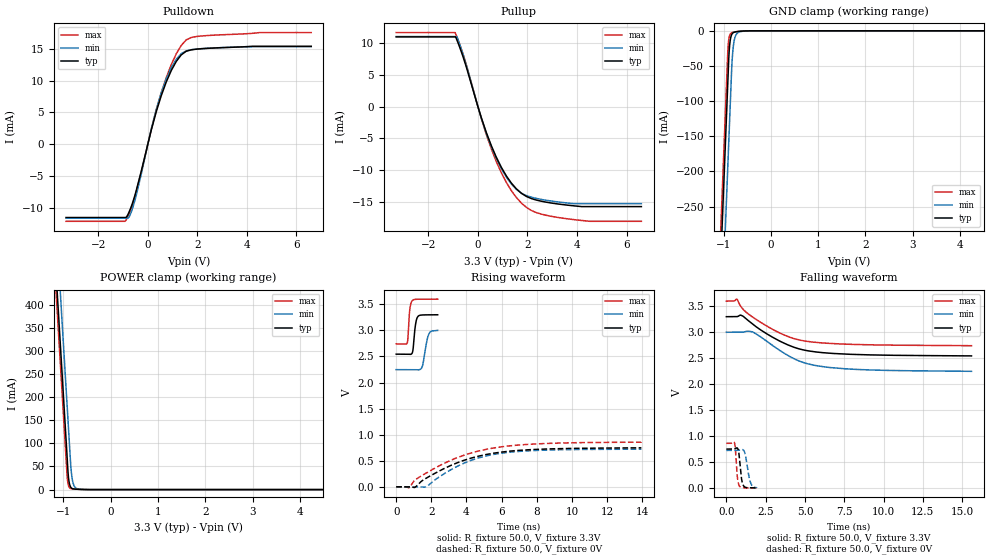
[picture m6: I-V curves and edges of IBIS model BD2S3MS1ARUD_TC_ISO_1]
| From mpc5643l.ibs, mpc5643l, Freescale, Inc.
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| *** New cell (Generated with 5.14beta1 (Sep 20 2010 13:23:23))
[Model]   BD2S3MS1ARUD_TC_ISO_1
Model_type I/O
Polarity   Non-Inverting
Enable   Active-Low
| CAP_THRESHOLD on pad pad is "CMOS" :
| Rising=10.0% of VDDE1   Falling=90.0% of VDDE1
| C_comp min and max val. don't necessarily correlate with the min and max pvt
| but are the smallest and greatest pad capacitance found.
| var   typ   min   max
C_comp   1.63948pF  1.52802pF  1.77729pF
Vinl = 1.05V | Dummy value overriden by next lines
Vinh = 2.34V | Dummy value overriden by next lines
Vmeas = 1.65V   | Reference voltage for timing measurements
Cref  = 25.0pF   | Timing specification test load capacitance value
Rref  = 1.0MOhm   | Timing specification test load resistance value
Vref  = 1.65V   | Timing specification test load voltage
[Model Spec]
| TIME_THRESHOLD on pin ipp_ind is "CORE" :
| Rising=40.0% of VDD   Falling=60.0% of VDD
Vinl 1.30950V 1.19650V 1.40650V
Vinh 1.89650V 1.72150V 2.04550V
| variable   typ   min   max
[Temperature Range] 25.0 150.0 -40.0
| variable   typ   min   max
[Voltage Range] 3.3V 3.0V 3.6V
| variable   typ   min   max
[POWER Clamp Reference] 3.3V 3.0V 3.6V
| variable   typ   min   max
[GND Clamp Reference] 0V 0V 0V
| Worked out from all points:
|   slope of the pulldown table from 0 to 0.495 V, typ, clamps not added: 70.3 ohm
|   slope of the pullup table from 0 to 0.495 V, typ, clamps not added: 86.8 ohm
|   GND clamp passes 1 mA (typ) near -0.70 V on its own axis
|   POWER clamp passes 1 mA (typ) near -0.74 V on its own axis
|   rising waveform, R_fixture 50.0, V_fixture 3.3V: 20-80 % time 140ps typ, 232ps min, 105ps max; typ from 2.54 V to 3.3 V
|   falling waveform, R_fixture 50.0, V_fixture 3.3V: 20-80 % time 2.75ns typ, 2.63ns min, 2.85ns max; typ from 3.3 V to 2.54 V
|   rising waveform, R_fixture 50.0, V_fixture 0V: 20-80 % time 3.19ns typ, 2.7ns min, 3.44ns max; typ from 0 V to 0.748 V
|   falling waveform, R_fixture 50.0, V_fixture 0V: 20-80 % time 157ps typ, 248ps min, 123ps max; typ from 0.748 V to 0 V
[POWER Clamp]
-3.3V     4.118A     4.23A      4.076A
-1.21V    564.8mA    676.6mA    523.5mA
-1.14V    445.8mA    557.6mA    404.5mA
-1.07V    326.8mA    438.6mA    285.5mA
-1V       207.8mA    319.6mA    166.5mA
-920mV    71.78mA    183.6mA    30.49mA
-890mV    26.12mA    132.6mA    8.48mA
-850mV    6.633mA    64.57mA    2.709mA
-820mV    2.915mA    28.96mA    1.809mA
-790mV    1.645mA    13.25mA    1.441mA
-640mV    470.3uA    702.5uA    525.7uA
6.6V      0A         0A         0A
[GND Clamp]
-3.3V     -4.137A    -4.256A    -4.093A
-1.08V    -363.1mA   -482.3mA   -318.5mA
-920mV    -91.09mA   -210.3mA   -46.51mA
-910mV    -74.09mA   -193.3mA   -29.53mA
-900mV    -57.09mA   -176.3mA   -19.14mA
-880mV    -27.98mA   -142.3mA   -8.85mA
-860mV    -14.09mA   -108.3mA   -4.88mA
-820mV    -4.49mA    -44.02mA   -2.507mA
-790mV    -2.505mA   -20.34mA   -1.929mA
-750mV    -1.544mA   -7.742mA   -1.439mA
-580mV    -311.3uA   -595.3uA   -220.1uA
6.6V      3.126nA    968.2nA    21.28pA
| variable   typ   min   max
[Pullup Reference] 3.3V 3.0V 3.6V
| variable   typ   min   max
[Pulldown Reference] 0V 0V 0V
[Pullup]
-3.3V     11.03mA    11.09mA    11.72mA
-920mV    11.03mA    11.09mA    11.72mA
-850mV    10.55mA    11.09mA    11.04mA
-700mV    9.003mA    9.426mA    9.462mA
-470mV    6.281mA    6.567mA    6.637mA
140mV     -1.782mA   -1.838mA   -1.918mA
740mV     -7.979mA   -8.178mA   -8.659mA
1.35V     -12.08mA   -12.23mA   -13.28mA
1.96V     -14.21mA   -14.08mA   -15.93mA
2.57V     -14.96mA   -14.67mA   -17mA
3.78V     -15.65mA   -15.31mA   -17.82mA
6.6V      -15.81mA   -15.33mA   -18.13mA
[Pulldown]
-3.3V     -11.52mA   -11.61mA   -12.11mA
-890mV    -11.52mA   -11.61mA   -11.99mA
-740mV    -10.5mA    -11.31mA   -10.8mA
-550mV    -8.419mA   -9.215mA   -8.653mA
-270mV    -4.331mA   -4.79mA    -4.454mA
140mV     2.228mA    2.408mA    2.326mA
340mV     5.098mA    5.459mA    5.363mA
740mV     9.751mA    10.23mA    10.43mA
1.15V     13.03mA    13.37mA    14.23mA
1.55V     14.63mA    14.7mA     16.41mA
2.54V     15.11mA    15.12mA    17.13mA
6.6V      15.41mA    15.34mA    17.57mA
[Ramp]
dV/dt_r 448.50528mV/3.19466ns 433.17622mV/2.69643ns 515.10028mV/3.44347ns
dV/dt_f 453.48808mV/2.74568ns 451.77072mV/2.63236ns 515.29527mV/2.85052ns
R_load = 50.0
| Removed startup time: 0s 0s 0s  .
| Removed end time: 2.359ns.
[Rising Waveform]
R_fixture   = 50.0
V_fixture   = 3.3V
V_fixture_min = 3.0V
V_fixture_max = 3.6V
0s        2.544V     2.247V     2.741V
627ps     2.544V     2.247V     2.758V
666ps     2.544V     2.247V     2.847V
773ps     2.54V      2.247V     3.399V
925ps     2.578V     2.247V     3.575V
1.088ns   3.088V     2.247V     3.595V
1.219ns   3.259V     2.243V     3.598V
1.491ns   3.296V     2.314V     3.599V
1.864ns   3.298V     2.934V     3.599V
2.361ns   3.3V       2.999V     3.6V
| Removed startup time: 0s 0s 0s  .
| Removed end time: 15.588ns.
[Falling Waveform]
R_fixture   = 50.0
V_fixture   = 3.3V
V_fixture_min = 3.0V
V_fixture_max = 3.6V
0s        3.3V       3V         3.6V
456ps     3.3V       3V         3.6V
663ps     3.301V     3V         3.638V
942ps     3.327V     3V         3.489V
1.662ns   3.16V      3.007V     3.295V
3.333ns   2.84V      2.663V     2.995V
4.746ns   2.67V      2.432V     2.844V
6.003ns   2.61V      2.342V     2.797V
7.926ns   2.575V     2.289V     2.767V
15.59ns   2.544V     2.247V     2.741V
| Removed startup time: 0s 0s 0s  .
| Removed end time: 13.947ns.
[Rising Waveform]
R_fixture   = 50.0
V_fixture   = 0V
V_fixture_min = 0V
V_fixture_max = 0V
0s        12.1nV     412.9nV    11.83nV
720ps     658.4uV    -790.7nV   -19.83mV
1.053ns   -12.65mV   242.6uV    123mV
1.656ns   155mV      -4.777mV   253.8mV
3.465ns   458.9mV    391.6mV    558.2mV
4.197ns   543.9mV    499.6mV    641.9mV
5.247ns   627.1mV    601.1mV    726.7mV
6.441ns   682.9mV    663.1mV    784.8mV
8.118ns   719.9mV    699.5mV    825.1mV
13.95ns   747.5mV    722mV      858.5mV
| Removed startup time: 0s 0s 0s  .
| Removed end time: 1.931ns.
[Falling Waveform]
R_fixture   = 50.0
V_fixture   = 0V
V_fixture_min = 0V
V_fixture_max = 0V
0s        747.5mV    722mV      858.5mV
524ps     751.8mV    721.8mV    860.5mV
579ps     759.9mV    721.7mV    745.9mV
699ps     767.1mV    721.8mV    215.3mV
824ps     599mV      727.5mV    37.53mV
953ps     203mV      739.1mV    6.896mV
1.085ns   44.99mV    729mV      1.666mV
1.215ns   10.01mV    630.8mV    671.6uV
1.545ns   1.012mV    97.51mV    346.3uV
1.933ns   165.9uV    284.1uV    131.2uV
